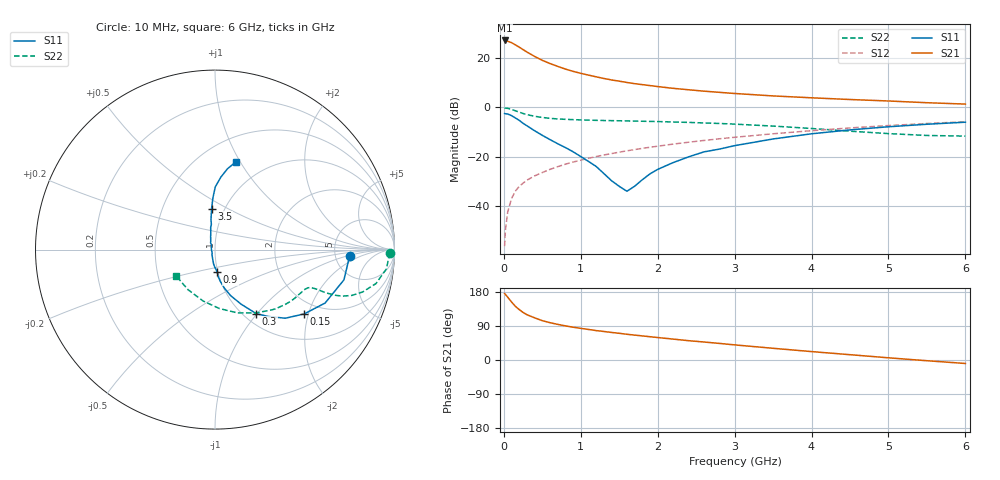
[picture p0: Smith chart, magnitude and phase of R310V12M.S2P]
! SIEMENS Small Signal Semiconductors
! BFR181
! Si NPN RF Bipolar Junction Transistor in SOT23
! VCE = 10 V  IC = 12 mA
! Common Emitter S-Parameters:  May  1996
# GHz  S  MA  R  50
!  f  S11  S21  S12  S22
! GHz  MAG  ANG  MAG  ANG  MAG  ANG  MAG  ANG
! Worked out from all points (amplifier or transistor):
!   36 points, 10 MHz to 6 GHz, reference 50 ohm
!   highest |S21| = 27.3 dB at 10 MHz (marker M1)
!   |S21| within 3 dB of that: start of sweep to 213.5 MHz
!   unconditionally stable (mu >= 1): 839.7 MHz to 2.848 GHz
!   at 250 MHz: K = 0.62, MSG = 27.2 dB, |S12| = -30.8 dB
!   at 1.4 GHz: K = 1.05, MAG = 13.7 dB, |S12| = -18.8 dB
!   at 6 GHz: K = 0.87, MSG = 3.6 dB, |S12| = -5.8 dB
!   S11 on the Smith chart (normalised r, x): 10 MHz: 6.96, -1.06; 150 MHz: 1.64, -1.88; 300 MHz: 1.14, -0.99; 900 MHz: 0.99, -0.25; 3.5 GHz: 0.87, +0.42; 6 GHz: 0.73, +0.96
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0.01  0.7537 -2.5  23.17 175.5  0.0015 76.3  0.9762 -1.1
0.02  0.7459 -5.0  22.81 173.1  0.0031 83.0  0.9693 -2.6
0.05  0.7379 -13.2  22.28 165.8  0.0074 84.8  0.9611 -6.4
0.1  0.6818 -25.9  20.89 153.2  0.014 76.1  0.9169 -11.9
0.15  0.6126 -35.8  18.84 141.7  0.0198 72.4  0.856 -16.0
0.2  0.5474 -44.3  16.91 133.1  0.0248 71.5  0.8044 -18.5
0.25  0.4759 -51.5  15.09 125.5  0.0288 69.9  0.7547 -20.1
0.3  0.4246 -57.2  13.47 119.5  0.0331 69.9  0.7155 -20.8
0.4  0.3363 -64.5  10.96 111.3  0.0405 68.8  0.6626 -21.3
0.5  0.271 -71.2  9.123 103.8  0.0474 69.6  0.6262 -21.3
0.6  0.2219 -76.2  7.85 98.5  0.0549 69.8  0.6015 -21.3
0.7  0.183 -80.1  6.866 94.0  0.0623 70.4  0.5846 -21.5
0.9  0.1255 -84.1  5.442 86.5  0.0775 70.4  0.5657 -22.0
1.1  0.0798 -95.8  4.564 80.6  0.0924 70.0  0.5527 -23.2
1.3  0.0452 -108.9  3.897 75.3  0.1078 69.6  0.543 -24.7
1.6  0.0197 -178.0  3.232 67.9  0.1312 68.2  0.532 -27.6
2.2  0.0754 108.8  2.456 55.2  0.1796 64.5  0.5072 -35.1
2.8  0.1419 98.2  2.037 43.8  0.2301 59.9  0.4728 -44.2
3.5  0.2286 94.8  1.72 30.9  0.2915 53.5  0.4182 -57.7
4.5  0.35 89.7  1.453 14.0  0.3836 42.9  0.3294 -85.7
5.5  0.4558 81.2  1.251 -1.9  0.4719 30.7  0.2692 -124.0
6  0.5018 76.7  1.173 -9.2  0.5131 24.0  0.2613 -146.0
